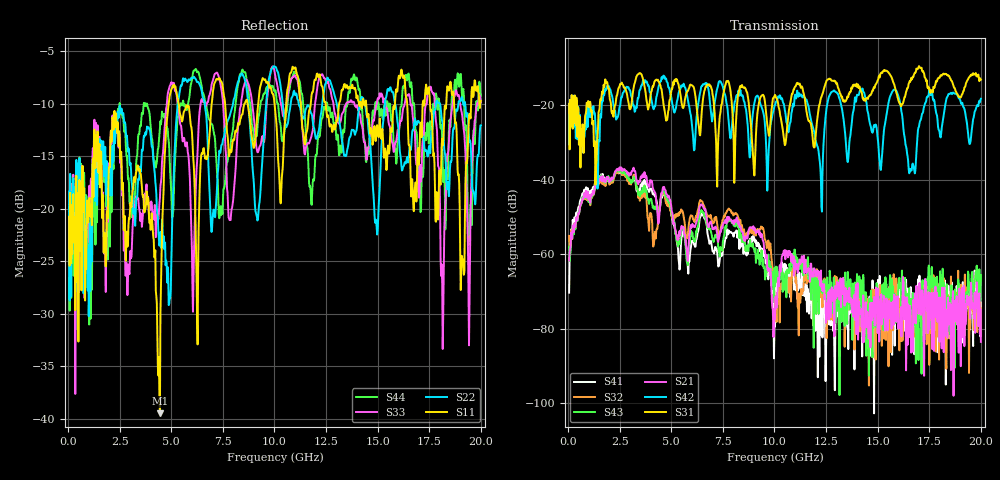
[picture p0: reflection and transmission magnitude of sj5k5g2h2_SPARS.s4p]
! FILE: E:\users\goganessyan\GBX_Backplane\FR408_backplane\1m_INBOUND_FEXT\sj5k5g2h2_SPARS.s4p
# MHZ S RI R 50.00
! FREQ  S11  S12  S13  S14
!  S21  S22  S23  S24
!  S31  S32  S33  S34
!  S41  S42  S43  S44
!  REAL  IMAG  REAL  IMAG  REAL  IMAG  REAL  IMAG
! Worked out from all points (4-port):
!   799 points, 50 MHz to 20 GHz, reference 50 ohm
!   strongest paths, dB at 50 MHz, 5.025 GHz, 10.03 GHz, 15.03 GHz, 20 GHz:
!     S31: -19.7, -15.5, -17.3, -13.1, -13.2
!     S42: -19.6, -18.8, -20.0, -30.1, -18.3
!     S21: -61.7, -48.6, -77.5, -69.2, -83.6
!     S43: -58.0, -48.8, -68.7, -73.7, -65.6
!     S32: -55.1, -49.7, -73.5, -78.7, -75.5
!     S41: -70.4, -49.9, -79.4, -66.9, -73.0
!   lowest |S11| = -39.5 dB at 4.45 GHz (marker M1), VSWR 1.02, Z = 51 - j0.239 ohm
!   |S11| at or under -10 dB: start of sweep to 4.874 GHz; 5.355 GHz to 6.957 GHz (1.602 GHz wide, 26 % of centre); 14.44 GHz to 15.84 GHz (1.395 GHz wide, 9.21 % of centre)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
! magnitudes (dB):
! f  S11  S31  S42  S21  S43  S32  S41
! 50 MHz  -20.8  -19.7  -19.6  -61.7  -58.0  -55.1  -70.4
! 1.45 GHz  -13.3  -26.1  -39.2  -41.1  -40.6  -41.3  -40.2
! 4.45 GHz  -39.5  -14.3  -13.8  -47.6  -47.0  -46.7  -47.7
! 5.075 GHz  -8.3  -14.5  -20.2  -50.1  -50.3  -49.7  -51.6
! 12.25 GHz  -8.0  -18.1  -40.0  -64.4  -66.6  -67.8  -73.2
! 12.82 GHz  -12.5  -13.5  -16.3  -72.2  -75.2  -76.5  -71.6
! 20 GHz  -9.7  -13.2  -18.3  -83.6  -65.6  -75.5  -73.0
